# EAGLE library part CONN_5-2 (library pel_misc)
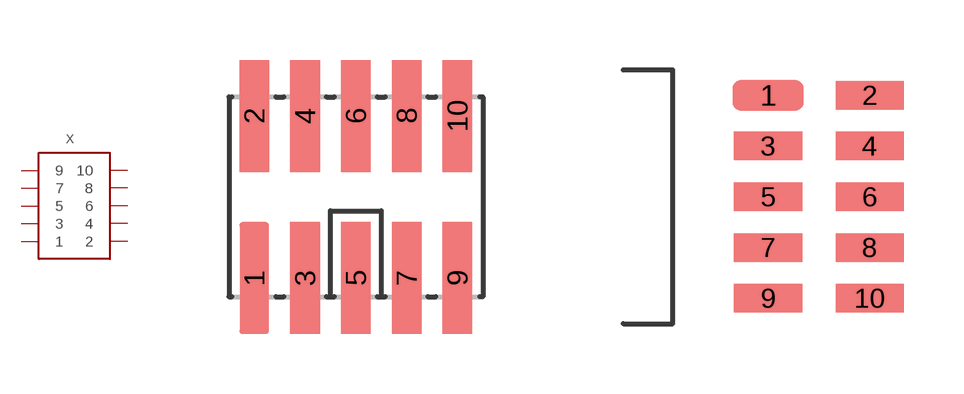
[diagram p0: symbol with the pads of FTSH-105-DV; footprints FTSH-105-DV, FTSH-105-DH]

Designator prefix X

## CONN_5-2-FTSH-V  [FTSH-105-DV]
1  1
2  2
3  3
4  4
5  5
6  6
7  7
8  8
9  9
10  10

## CONN_5-2-FTSH-H  [FTSH-105-DH]
Pads as for FTSH-105-DV

## CONN_5-2  [FTSH-105-D]
Pads as for FTSH-105-DV

## Footprint FTSH-105-DV (pad centres in mm)
smd 0.74 x 2.8: 1 -2.54,-2.03; 2 -2.54,2.03; 3 -1.27,-2.03; 4 -1.27,2.03; 5 0,-2.03; 6 0,2.03; 7 1.27,-2.03; 8 1.27,2.03; 9 2.54,-2.03; 10 2.54,2.03

## Footprint FTSH-105-DH (pad centres in mm)
smd 1.78 x 0.76: 1 -1.27,2.54
smd 1.702 x 0.711: 2 1.27,2.54; 3 -1.27,1.27; 4 1.27,1.27; 5 -1.27,0; 6 1.27,0; 7 -1.27,-1.27; 8 1.27,-1.27; 9 -1.27,-2.54; 10 1.27,-2.54

## Footprint FTSH-105-D (pad centres in mm)
drill 0.71 pad 1.016 octagon: 1 -2.54,-0.635; 2 -2.54,0.635; 3 -1.27,-0.635; 4 -1.27,0.635; 5 0,-0.635; 6 0,0.635; 7 1.27,-0.635; 8 1.27,0.635; 9 2.54,-0.635; 10 2.54,0.635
